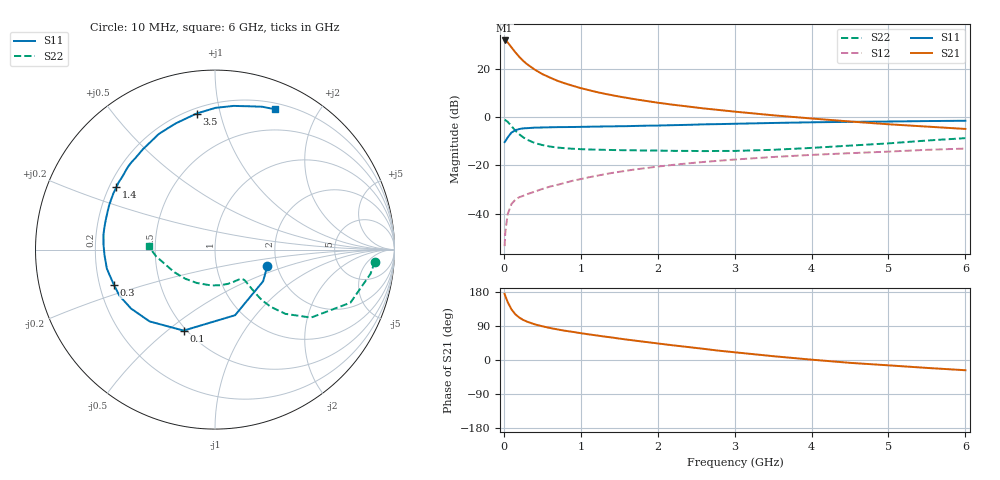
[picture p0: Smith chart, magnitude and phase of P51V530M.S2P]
! SIEMENS Small Signal Semiconductors
! BFP183
! Si NPN RF Bipolar Junction Transistor in SOT143
! VCE = 1.5 V  IC = 30 mA
! Common Emitter S-Parameters:  March  1996
# GHz  S  MA  R  50
!  f  S11  S21  S12  S22
! GHz  MAG  ANG  MAG  ANG  MAG  ANG  MAG  ANG
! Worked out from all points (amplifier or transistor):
!   36 points, 10 MHz to 6 GHz, reference 50 ohm
!   highest |S21| = 32.0 dB at 10 MHz (marker M1)
!   |S21| within 3 dB of that: start of sweep to 102.7 MHz
!   unconditionally stable (mu >= 1): start of sweep to 11.57 MHz; 422.3 MHz to end of sweep
!   at 250 MHz: K = 0.74, MSG = 28.1 dB, |S12| = -32.7 dB
!   at 1.4 GHz: K = 1.34, MAG = 12.7 dB, |S12| = -23.1 dB
!   at 6 GHz: K = 1.07, MAG = 2.5 dB, |S12| = -13.0 dB
!   S11 on the Smith chart (normalised r, x): 10 MHz: 1.78, -0.36; 100 MHz: 0.48, -0.57; 300 MHz: 0.26, -0.16; 1.4 GHz: 0.23, +0.28; 3.5 GHz: 0.23, +0.85; 6 GHz: 0.26, +1.48
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0.01  0.3056 -17.3  39.73 174.3  0.0021 74.5  0.8931 -4.3
0.02  0.3209 -33.3  39.46 168.7  0.0042 80.1  0.8766 -8.9
0.05  0.3824 -73.0  36.16 152.8  0.0097 70.8  0.8106 -21.4
0.1  0.484 -111.2  28.49 133.4  0.0159 54.3  0.6555 -35.3
0.15  0.5411 -132.3  22.48 120.5  0.0194 49.6  0.5308 -42.4
0.2  0.5715 -144.9  18.19 112.1  0.0219 48.8  0.4459 -45.7
0.25  0.5909 -154.1  15.07 105.9  0.0233 48.2  0.3869 -47.1
0.3  0.5964 -160.6  12.83 101.3  0.0252 47.9  0.345 -47.2
0.4  0.6117 -169.9  9.877 94.2  0.0285 51.1  0.2941 -46.8
0.5  0.6164 -177.0  7.953 89.0  0.0325 51.3  0.2657 -46.4
0.6  0.622 177.3  6.712 84.5  0.0364 53.3  0.2476 -46.0
0.7  0.627 172.3  5.729 80.6  0.0397 54.8  0.2354 -46.1
0.8  0.6286 168.6  5.058 77.1  0.0438 56.2  0.2281 -46.6
1.1  0.6393 157.4  3.699 67.7  0.0566 57.1  0.2149 -49.8
1.4  0.6502 147.6  2.908 59.5  0.0697 56.4  0.2098 -55.2
1.7  0.6631 138.9  2.388 51.3  0.0825 54.7  0.2068 -61.9
2.2  0.6885 125.7  1.832 38.7  0.103 50.8  0.2013 -75.2
2.8  0.7247 111.5  1.423 24.5  0.1255 45.0  0.2004 -94.3
3.5  0.7651 97.7  1.105 10.1  0.15 38.5  0.2118 -118.6
4.5  0.8073 82.6  0.821 -7.5  0.18 28.8  0.2589 -150.8
5.5  0.838 71.8  0.643 -20.9  0.2115 20.1  0.33 -173.4
6  0.8501 67.0  0.575 -27.0  0.2245 15.2  0.3698 177.2
